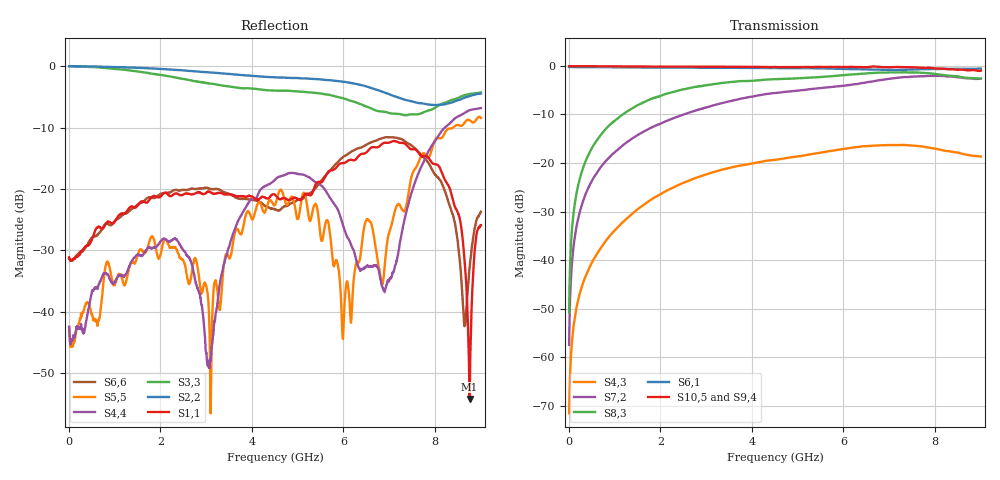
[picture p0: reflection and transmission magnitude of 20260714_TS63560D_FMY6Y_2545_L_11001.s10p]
# GHz S DB R 50
! CMT, SN0916, 25263762, 26.7.0
! Date: 15.07.2026 13:47:15
! Data: Format
! Freq S1.1:dB/Ang S1.2:dB/Ang S1.3:dB/Ang S1.4:dB/Ang S1.5:dB/Ang S1.6:dB/Ang S1.7:dB/Ang S1.8:dB/Ang S1.9:dB/Ang S1.10:dB/Ang
!  S2.1:dB/Ang S2.2:dB/Ang S2.3:dB/Ang S2.4:dB/Ang S2.5:dB/Ang S2.6:dB/Ang S2.7:dB/Ang S2.8:dB/Ang S2.9:dB/Ang S2.10:dB/Ang
!  S3.1:dB/Ang S3.2:dB/Ang S3.3:dB/Ang S3.4:dB/Ang S3.5:dB/Ang S3.6:dB/Ang S3.7:dB/Ang S3.8:dB/Ang S3.9:dB/Ang S3.10:dB/Ang
!  S4.1:dB/Ang S4.2:dB/Ang S4.3:dB/Ang S4.4:dB/Ang S4.5:dB/Ang S4.6:dB/Ang S4.7:dB/Ang S4.8:dB/Ang S4.9:dB/Ang S4.10:dB/Ang
!  S5.1:dB/Ang S5.2:dB/Ang S5.3:dB/Ang S5.4:dB/Ang S5.5:dB/Ang S5.6:dB/Ang S5.7:dB/Ang S5.8:dB/Ang S5.9:dB/Ang S5.10:dB/Ang
!  S6.1:dB/Ang S6.2:dB/Ang S6.3:dB/Ang S6.4:dB/Ang S6.5:dB/Ang S6.6:dB/Ang S6.7:dB/Ang S6.8:dB/Ang S6.9:dB/Ang S6.10:dB/Ang
!  S7.1:dB/Ang S7.2:dB/Ang S7.3:dB/Ang S7.4:dB/Ang S7.5:dB/Ang S7.6:dB/Ang S7.7:dB/Ang S7.8:dB/Ang S7.9:dB/Ang S7.10:dB/Ang
!  S8.1:dB/Ang S8.2:dB/Ang S8.3:dB/Ang S8.4:dB/Ang S8.5:dB/Ang S8.6:dB/Ang S8.7:dB/Ang S8.8:dB/Ang S8.9:dB/Ang S8.10:dB/Ang
!  S9.1:dB/Ang S9.2:dB/Ang S9.3:dB/Ang S9.4:dB/Ang S9.5:dB/Ang S9.6:dB/Ang S9.7:dB/Ang S9.8:dB/Ang S9.9:dB/Ang S9.10:dB/Ang
!  S10.1:dB/Ang S10.2:dB/Ang S10.3:dB/Ang S10.4:dB/Ang S10.5:dB/Ang S10.6:dB/Ang S10.7:dB/Ang S10.8:dB/Ang S10.9:dB/Ang S10.10:dB/Ang
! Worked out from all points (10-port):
!   2001 points, 10 MHz to 9 GHz, reference 50 ohm
!   strongest paths, dB at 10 MHz, 2.257 GHz, 4.505 GHz, 6.753 GHz, 9 GHz:
!     S10,5: -0.1, -0.2, -0.2, -0.2, -1.0
!     S9,4: -0.1, -0.2, -0.4, -0.4, -1.5
!     S6,1: -0.2, -0.4, -0.5, -0.8, -0.6
!     S8,3: -50.7, -5.5, -2.8, -1.4, -2.6
!     S7,2: -57.4, -10.9, -5.6, -3.0, -2.7
!     S4,3: -71.5, -25.2, -19.3, -16.4, -18.7
!   lowest |S11| = -54.2 dB at 8.753 GHz (marker M1), VSWR 1.00, Z = 50 - j0.193 ohm
!   |S11| at or under -10 dB: start of sweep to end of sweep
